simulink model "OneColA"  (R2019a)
settings: Solver=ode15s  StartTime=0.0  StopTime=tend  RelTol=1e-3
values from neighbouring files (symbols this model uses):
  Extract_J = zeros(83,1)'    [Simulate1Col.m]    (also in Simulate1Col_OL.m; Simulate1Col_R1.m; Simulate1Col_R2.m)
  Extract_xB = zeros(82,1)'    [Simulate1Col.m]    (also in Simulate1Col_OL.m; Simulate1Col_R1.m; Simulate1Col_R2.m)
  Extract_xD = zeros(82,1)'    [Simulate1Col.m]    (also in Simulate1Col_OL.m; Simulate1Col_R1.m; Simulate1Col_R2.m)
  F0 = 1    [colamod.m]    (also in ColumnA_simulation.m; Simulate1Col.m = F; Simulate1Col_OL.m = F; Simulate1Col_R1.m = F)
  F0step = 0.05    [Simulate1Col.m]    (also in Simulate1Col_OL.m = 1*F0*.1; Simulate1Col_R1.m; Simulate1Col_R2.m = 0.15)
  F0step_t = 10    [Simulate1Col.m]    (also in Simulate1Col_OL.m; Simulate1Col_R1.m; Simulate1Col_R2.m)
  LT0 = u_opt(1)    [Simulate1Col.m]    (also in Simulate1Col_OL.m; Simulate1Col_R1.m; Simulate1Col_R2.m)
  LTstep = 0*LT0*.2    [Simulate1Col_OL.m]
  LTstep_t = 10    [Simulate1Col_OL.m]
  pV0 = pV    [Simulate1Col.m]    (also in Simulate1Col_OL.m; Simulate1Col_R1.m; Simulate1Col_R2.m)
  pVstep = 0.02    [Simulate1Col.m]    (also in Simulate1Col_OL.m = 0*(0.13-pV0); Simulate1Col_R1.m; Simulate1Col_R2.m = 0.06)
  pVstept = 50    [Simulate1Col.m]    (also in Simulate1Col_OL.m; Simulate1Col_R1.m; Simulate1Col_R2.m)
  qF = U(7)    [colamod.m]    (also in ColumnA_simulation.m; Simulate1Col.m = 1; Simulate1Col_OL.m = 1; Simulate1Col_R1.m = 1)
  VB0 = u_opt(2)    [Simulate1Col.m]    (also in Simulate1Col_OL.m; Simulate1Col_R1.m; Simulate1Col_R2.m)
  VBstep = 0*VB0*.1    [Simulate1Col_OL.m]
  VBstep_t = 10    [Simulate1Col_OL.m]
  x0 = 0.5*ones(1,82)'    [col_obj.m]    (also in Simulate1Col.m = x; Simulate1Col_OL.m = x; Simulate1Col_R1.m = x; Simulate1Col_R2.m = x)
  zF = U(6)    [colamod.m]    (also in ColumnA_simulation.m; Simulate1Col.m = 0.5; Simulate1Col_OL.m = 0.5; Simulate1Col_R1.m = 0.5)
undefined symbols (not defined in the file or in its folder): ColumnA_simulation, extract

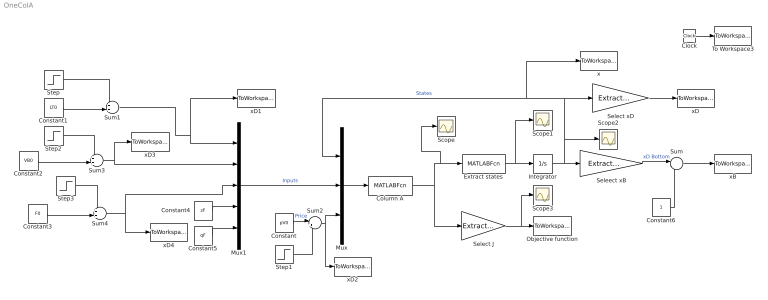
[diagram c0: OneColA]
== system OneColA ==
  Clock : Clock
  Column A : MATLABFcn  MATLABFcn=ColumnA_simulation(u)  OutputDimensions=83
  Constant : Constant  Value=pV0
  Constant1 : Constant  Value=LT0
  Constant2 : Constant  Value=VB0
  Constant3 : Constant  Value=F0
  Constant4 : Constant  Value=zF
  Constant5 : Constant  Value=qF
  Constant6 : Constant
  Extract states : MATLABFcn  MATLABFcn=extract(u)  OutputDimensions=82
  Integrator : Integrator  InitialCondition=x0
  Mux : Mux  Inputs=3
  Mux1 : Mux  Inputs=5
  Objective function : ToWorkspace  VariableName=Jactual  SampleTime=-1
  Scope{,1..3} (4 alike) : Scope
  Select J : Gain  Gain=Extract_J  Multiplication=Matrix(K*u)
  Select xD : Gain  Gain=Extract_xD  Multiplication=Matrix(K*u)
  Seleect xB : Gain  Gain=Extract_xB  Multiplication=Matrix(K*u)
  Step : Step  Time=LTstep_t  After=LTstep  SampleTime=0
  Step1 : Step  Time=pVstept  After=pVstep  SampleTime=0
  Step2 : Step  Time=VBstep_t  After=VBstep  SampleTime=0
  Step3 : Step  Time=F0step_t  After=F0step  SampleTime=0
  Sum : Sum  Inputs=|-+
  Sum1 : Sum  Inputs=++|
  Sum2 : Sum  Inputs=|++
  Sum3 : Sum  Inputs=++|
  Sum4 : Sum  Inputs=++|
  To Workspace3 : ToWorkspace  VariableName=time  SampleTime=-1
  x : ToWorkspace  VariableName=States  SampleTime=-1
  xB : ToWorkspace  VariableName=xB  SampleTime=-1
  xD : ToWorkspace  VariableName=xD  SampleTime=-1
  xD1 : ToWorkspace  VariableName=LT  SampleTime=-1
  xD2 : ToWorkspace  VariableName=pV  SampleTime=-1
  xD3 : ToWorkspace  VariableName=VB  SampleTime=-1
  xD4 : ToWorkspace  VariableName=Fin  SampleTime=-1
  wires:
  Mux/1 -> Column A/1
  Mux1/1 -> Mux/2  "Inputs"
  Constant4/1 -> Mux1/4
  Constant5/1 -> Mux1/5
  Column A/1 -> Select J/1, Extract states/1, Scope/1
  Extract states/1 -> Scope1/1, Integrator/1
  Integrator/1 -> Seleect xB/1, Select xD/1, x/1, Mux/1, Scope2/1  "States"
  Select xD/1 -> xD/1
  Select J/1 -> Scope3/1, Objective function/1
  Clock/1 -> To Workspace3/1
  Seleect xB/1 -> Sum/1  "xD Bottom"
  Sum/1 -> xB/1
  Constant6/1 -> Sum/2
  Sum1/1 -> xD1/1, Mux1/1
  Constant1/1 -> Sum1/2
  Sum2/1 -> xD2/1, Mux/3
  Constant/1 -> Sum2/1  "Price"
  Constant2/1 -> Sum3/2
  Sum3/1 -> Mux1/2, xD3/1
  Step/1 -> Sum1/1
  Step2/1 -> Sum3/1
  Constant3/1 -> Sum4/2
  Sum4/1 -> xD4/1, Mux1/3
  Step3/1 -> Sum4/1
  Step1/1 -> Sum2/2
